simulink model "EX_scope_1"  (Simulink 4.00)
settings: Solver=ode45  StartTime=0.0  StopTime=3.99  FixedStep=0.1  MaxStep=0.1  MinStep=0.01  RelTol=1e-3

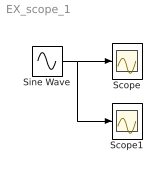
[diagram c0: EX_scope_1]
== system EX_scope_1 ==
  Scope : Scope
  Scope1 : Scope
  Sine Wave : Sin  SineType=Time-based  Amplitude=1  Bias=0  Frequency=5  Phase=0  Samples=10  SampleTime=0
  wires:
  Sine Wave/1 -> Scope/1, Scope1/1
